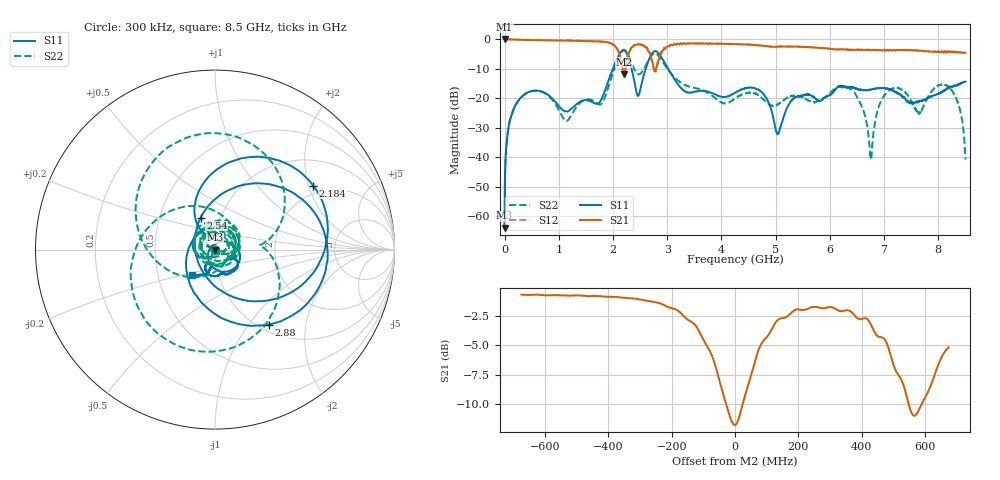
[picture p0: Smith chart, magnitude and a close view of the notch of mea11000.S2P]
!Agilent Technologies,E5071B,MY42402595,A.08.01
!Date: Tue Jan 02 09:06:34 2001
!Data & Calibration Information:
!Freq	S11:SOLT2(ON)	S21:SOLT2(ON)	S12:SOLT2(ON)	S22:SOLT2(ON)
# Hz S dB R 50
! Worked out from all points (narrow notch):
!   1601 points, 300 kHz to 8.5 GHz, reference 50 ohm
!   highest |S21| = 0.03 dB at 300 kHz (marker M1); lowest = -11.8 dB at 2.205 GHz (marker M2)
!   notch at M2: 9.3 dB deep, 112 MHz wide at half that depth
!   lowest |S11| = -63.8 dB at 300 kHz (marker M3), VSWR 1.00, Z = 50.1 - j0.0218 ohm
!   |S11| at or under -10 dB: start of sweep to 1.998 GHz; 2.343 GHz to 2.603 GHz (259.9 MHz wide, 10.5 % of centre); 3.016 GHz to end of sweep
!   |S22| runs from -63.9 to -3.7 dB; largest |S21 - S12| = 0.056
!   S11 on the Smith chart (normalised r, x): 300 kHz: 1.00, -0.00; 2.184 GHz: 1.73, +2.15; 2.54 GHz: 0.80, +0.30; 2.88 GHz: 1.11, -1.26; 8.5 GHz: 0.74, -0.22
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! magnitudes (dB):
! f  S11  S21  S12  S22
! 300 kHz  -63.8  0.0  0.0  -63.9
! 74.67 MHz  -29.6  -0.1  -0.1  -29.7
! 281.9 MHz  -20.1  -0.2  -0.2  -20.2
! 1.419 GHz  -21.0  -0.6  -0.6  -21.2
! 1.796 GHz  -20.0  -0.8  -0.8  -21.7
! 2.184 GHz  -3.7  -10.6  -10.8  -3.9
! 2.205 GHz  -3.7  -11.8  -11.4  -3.7
! 2.449 GHz  -19.0  -1.7  -1.9  -11.7
! 2.54 GHz  -14.2  -2.1  -2.0  -11.0
! 2.837 GHz  -4.7  -7.4  -7.1  -5.6
! 2.88 GHz  -5.8  -5.2  -4.4  -6.7
! 3.342 GHz  -17.9  -1.6  -1.5  -15.7
! 4.25 GHz  -18.1  -1.7  -1.7  -20.1
! 4.728 GHz  -17.7  -2.1  -2.1  -19.6
! 5.036 GHz  -32.3  -2.6  -2.6  -22.1
! 5.669 GHz  -19.3  -2.7  -2.8  -21.2
! 6.407 GHz  -16.3  -3.7  -3.6  -17.1
! 6.758 GHz  -17.0  -3.6  -3.6  -40.8
! 7.087 GHz  -17.0  -3.9  -3.7  -17.5
! 7.639 GHz  -21.1  -3.9  -3.9  -25.2
! 8.181 GHz  -16.7  -4.1  -4.3  -16.0
! 8.5 GHz  -14.4  -4.6  -4.6  -40.8
